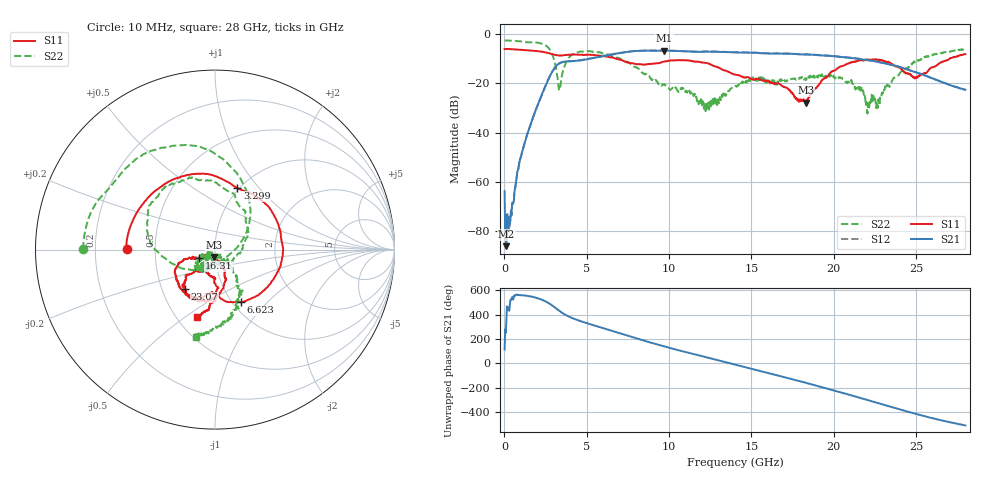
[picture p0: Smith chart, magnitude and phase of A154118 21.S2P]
!  2-Port S-parameters saved by WinCal
! VAR MeasName=S-Parameters (CALIBRATED_DATA) read from VNA (N5230A)
! VAR MeasDate=2015-9-10 14:35:59
! VAR NAME=A154118 21
! VAR FILENAME=A154118 21.S2P
! VAR DATE=2015-9-10 14:35:59
! VAR PHYS_PORTS=1,2
# Hz S DB R 50
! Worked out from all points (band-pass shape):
!   801 points, 10 MHz to 28 GHz, reference 50 ohm
!   highest |S21| = -6.77 dB at 9.702 GHz (marker M1); lowest = -86.0 dB at 115 MHz (marker M2)
!   |S21| within 3 dB of the highest: 5.423 GHz to 21.03 GHz (15.61 GHz wide, 118 % of centre); 21.06867 GHz to 21.07349 GHz (4.817 MHz wide, 0.0229 % of centre)
!   lowest |S11| = -27.8 dB at 18.31 GHz (marker M3), VSWR 1.08, Z = 49.4 - j4 ohm
!   |S11| at or under -10 dB: 6.77 GHz to 27.06 GHz (20.29 GHz wide, 120 % of centre)
!   |S22| runs from -32.3 to -2.7 dB; largest |S21 - S12| = 0.0082
!   S11 on the Smith chart (normalised r, x): 10 MHz: 0.34, +0.00; 3.299 GHz: 0.98, +0.78; 6.623 GHz: 1.09, -0.72; 16.31 GHz: 0.83, -0.08; 23.07 GHz: 0.65, -0.31; 28 GHz: 0.63, -0.56
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1e7  -6.16 179.6  -63.76 114.0  -81.23 97.5  -2.67 179.8
1.149625e8  -6.12 176.1  -86.02 -18.5  -74.05 -105.0  -2.69 177.2
4.2985e8  -6.21 165.5  -73.58 163.4  -73.29 160.7  -2.75 169.5
1.199575e9  -6.53 141.1  -44.87 -161.7  -44.88 -161.6  -3.30 150.6
2.424138e9  -7.39 98.3  -22.14 154.2  -22.11 154.4  -4.37 105.3
3.298825e9  -8.75 70.2  -12.07 75.1  -12.06 75.2  -22.07 -28.2
3.893612e9  -8.52 49.9  -11.13 25.9  -11.11 26.1  -9.83 -178.3
4.698325e9  -8.48 14.3  -10.65 -16.0  -10.62 -15.8  -7.13 143.9
6.622638e9  -9.71 -63.6  -8.23 -96.1  -8.15 -96.2  -9.26 82.0
9.351662e9  -11.90 -101.5  -6.86 153.5  -6.79 153.2  -20.41 -43.0
9.701538e9  -11.21 -105.0  -6.77 140.4  -6.74 139.9  -20.35 -69.8
1.229061e10  -11.85 -150.9  -7.17 49.9  -7.13 49.3  -29.21 -116.1
1.4005e10  -16.49 -162.6  -7.48 -9.3  -7.45 -9.9  -21.49 -104.2
1.631418e10  -20.04 -152.1  -7.96 -87.8  -7.95 -88.3  -19.16 -123.2
1.830846e10  -27.82 -96.1  -8.35 -158.9  -8.29 -158.9  -18.72 -119.0
1.869332e10  -23.33 -74.0  -8.44 -172.9  -8.46 -173.3  -16.75 -120.4
2.103749e10  -11.54 -88.6  -9.78 99.6  -9.66 98.6  -19.28 -151.1
2.208711e10  -10.39 -108.0  -10.69 58.8  -10.61 58.2  -28.11 -143.7
2.306676e10  -11.19 -127.5  -11.88 20.1  -11.86 19.4  -22.90 -46.0
2.334666e10  -11.56 -131.4  -12.32 9.3  -12.26 7.9  -20.83 -37.5
2.495609e10  -17.59 -114.2  -15.50 -52.3  -15.49 -53.1  -11.48 -58.2
2.8e10  -8.21 -104.6  -22.65 -148.8  -22.69 -150.0  -6.02 -102.2
